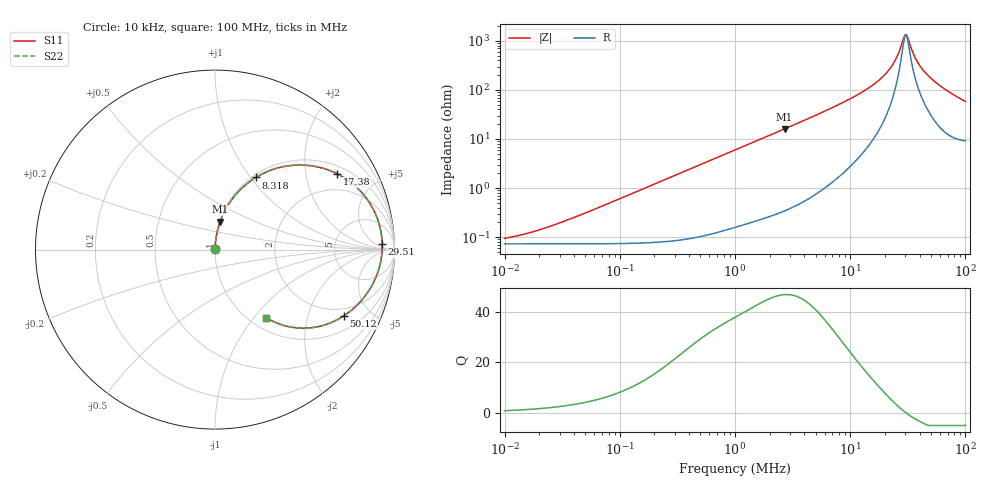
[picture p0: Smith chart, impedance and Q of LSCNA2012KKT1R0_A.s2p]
! LSCNA2012KKT1R0_A  S-PARAMETER MODEL  ( Standard Model )
! Model Generated by TAIYO YUDEN Corporation (http://www.ty-top.com)
! Version 1.0
! TAIYO YUDEN Control No. 170927
! Copyright(c) 2017 TAIYO YUDEN CO.,LTD. All Rights Reserved.
! Product Description (link to TY-COMPAS)
! https://ds.yuden.co.jp/TYCOMPAS/or/detail?pn=LSCNA2012KKT1R0MA&u=M
! Products Name : Inductors
! Characteristics :
!  Inductance : 1.0 [uH] , SRF(min) : - [Hz] , DC Resistance(max) : 90 [mOhm]
!  Rated Current : Saturation  3.6 [A] (dL = 30 [%]), Temp Rise  2.1 [A] (dT = 40 [degC])
!  Case Size : 2.0 x 1.25 / 0.079 x 0.049 [mm/inch] , Thickness : 1.0 / 0.039 [mm/inch]
!  (Conditions: Temperature = 25 [degC] , DC Bias Current = 0 [A])
! External Node Assignments :
!  1  o---GGG---o  2
! GND o---------o GND
! Frequency Range : 10kHz  -  100MHz  [ 402 STEP ]
# MHz S RI R 50
! Freq[MHz].  S11 Real  S11 Imag  S21 Real  S21 Imag  S12 Real  S12 Imag  S22 Real  S22 Imag
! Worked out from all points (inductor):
!   401 points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, 10 kHz to 100 MHz, reference 50 ohm
!   read as one part in series: L = 961 nH near 37.15 kHz
!   highest Q = 46.8 at 2.692 MHz (marker M1), where L = 951 nH
!   self-resonance near 30.47 MHz
!   S11 on the Smith chart (normalised r, x): 10 kHz: 1.00, +0.00; 8.318 MHz: 1.04, +1.06; 17.38 MHz: 1.28, +3.01; 29.51 MHz: 23, +11; 50.12 MHz: 1.61, -3.42; 100 MHz: 1.18, -1.15
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0.01  0.00073 0.000603  0.9993 -0.000603  0.9993 -0.000603  0.00073 0.000603
0.019498  0.000731 0.00118  0.9993 -0.00118  0.9993 -0.00118  0.000731 0.00118
0.046774  0.000739 0.00282  0.9993 -0.00282  0.9993 -0.00282  0.000739 0.00282
0.218776  0.000967 0.0132  0.999 -0.0132  0.999 -0.0132  0.000967 0.0132
1  0.00513 0.0595  0.9949 -0.0595  0.9949 -0.0595  0.00513 0.0595
2.691535  0.0284 0.1557  0.9716 -0.1557  0.9716 -0.1557  0.0284 0.1557
4.677351  0.0795 0.2589  0.9205 -0.2589  0.9205 -0.2589  0.0795 0.2589
6.309573  0.1386 0.3318  0.8614 -0.3318  0.8614 -0.3318  0.1386 0.3318
8.317638  0.2274 0.4021  0.7726 -0.4021  0.7726 -0.4021  0.2274 0.4021
12.58925  0.4469 0.4705  0.5531 -0.4705  0.5531 -0.4705  0.4469 0.4705
17.37801  0.68 0.4226  0.32 -0.4226  0.32 -0.4226  0.68 0.4226
21.87762  0.836 0.2956  0.164 -0.2956  0.164 -0.2956  0.836 0.2956
25.11886  0.9008 0.1826  0.0992 -0.1826  0.0992 -0.1826  0.9008 0.1826
29.51209  0.9315 0.0305  0.0685 -0.0305  0.0685 -0.0305  0.9315 0.0305
30.19952  0.9315 0.00829  0.0685 -0.00829  0.0685 -0.00829  0.9315 0.00829
31.62278  0.9281 -0.0358  0.0719 0.0358  0.0719 0.0358  0.9281 -0.0358
35.48134  0.9019 -0.1405  0.0981 0.1405  0.0981 0.1405  0.9019 -0.1405
39.81072  0.8545 -0.2325  0.1455 0.2325  0.1455 0.2325  0.8545 -0.2325
44.66836  0.7917 -0.3091  0.2083 0.3091  0.2083 0.3091  0.7917 -0.3091
50.11872  0.7178 -0.3692  0.2822 0.3692  0.2822 0.3692  0.7178 -0.3692
67.6083  0.5027 -0.4378  0.4973 0.4378  0.4973 0.4378  0.5027 -0.4378
100  0.2836 -0.3785  0.7164 0.3785  0.7164 0.3785  0.2836 -0.3785
